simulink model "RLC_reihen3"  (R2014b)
settings: Solver=ode45  StartTime=0.0  StopTime=0.005  RelTol=1e-3
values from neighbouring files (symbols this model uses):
  ampl_ug = 2    [RLC_reihen_1.m]    (also in RLC_reihen_3.m; RLC_reihen_4.m)
  C = [0 1 0 0;0 0 0 1]    [impuls_antw_zustand_1.m]    (also in impuls_antwort_1.m = 1e-07; impuls_antwort_2.m = 1e-07; impuls_antwort_3.m = 1e-07; impuls_antwort_4.m = 1e-07)
  f_ug = 1000    [RLC_reihen_1.m]    (also in RLC_reihen_3.m; RLC_reihen_4.m)
  i0 = 0    [RLC_reihen_1.m]    (also in RLC_reihen_3.m; RLC_reihen_4.m)
  L = 0.01    [impuls_antwort_1.m]    (also in impuls_antwort_2.m; impuls_antwort_3.m; impuls_antwort_4.m; RLC_reihen_1.m)
  phi_ug = pi/3    (= 1.0471975512)    [RLC_reihen_1.m]    (also in RLC_reihen_3.m; RLC_reihen_4.m)
  R = 50    [impuls_antwort_1.m]    (also in impuls_antwort_2.m; impuls_antwort_3.m; impuls_antwort_4.m; RLC_reihen_1.m)
  uc0 = -2    [RLC_reihen_1.m]    (also in RLC_reihen_3.m; RLC_reihen_4.m)

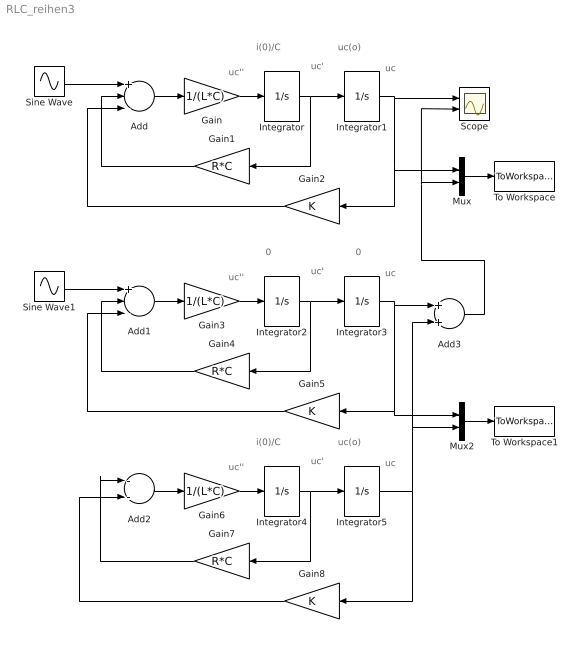
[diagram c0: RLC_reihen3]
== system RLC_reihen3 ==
  note: 0
  note: uc(o)
  note: i(0)/C
  note: uc''
  note: uc
  note: uc'
  note: 0
  note: uc''
  note: uc
  note: uc'
  note: uc(o)
  note: i(0)/C
  note: uc''
  note: uc
  note: uc'
  Add : Sum  Inputs=+--
  Add1 : Sum  Inputs=+--
  Add2 : Sum  Inputs=--
  Add3 : Sum
  Gain : Gain  Gain=1/(L*C)
  Gain1 : Gain  Gain=R*C
  Gain2 : Gain
  Gain3 : Gain  Gain=1/(L*C)
  Gain4 : Gain  Gain=R*C
  Gain5 : Gain
  Gain6 : Gain  Gain=1/(L*C)
  Gain7 : Gain  Gain=R*C
  Gain8 : Gain
  Integrator : Integrator  InitialCondition=i0/C
  Integrator1 : Integrator  InitialCondition=uc0
  Integrator2 : Integrator
  Integrator3 : Integrator
  Integrator4 : Integrator  InitialCondition=i0/C
  Integrator5 : Integrator  InitialCondition=uc0
  Mux : Mux  Inputs=2
  Mux2 : Mux  Inputs=2
  Scope : Scope  NumInputPorts=2
  Sine Wave : Sin  Amplitude=ampl_ug  Frequency=2*pi*f_ug  Phase=phi_ug  SampleTime=0
  Sine Wave1 : Sin  Amplitude=ampl_ug  Frequency=2*pi*f_ug  Phase=phi_ug  SampleTime=0
  To Workspace : ToWorkspace  VariableName=simout  SaveFormat=Timeseries  SampleTime=-1
  To Workspace1 : ToWorkspace  VariableName=simout1  SaveFormat=Timeseries  SampleTime=-1
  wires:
  Sine Wave/1 -> Add/1
  Add/1 -> Gain/1
  Gain/1 -> Integrator/1
  Integrator/1 -> Gain1/1, Integrator1/1
  Gain1/1 -> Add/2
  Gain2/1 -> Add/3
  Integrator1/1 -> Scope/1, Mux/1, Gain2/1
  Mux/1 -> To Workspace/1
  Sine Wave1/1 -> Add1/1
  Add1/1 -> Gain3/1
  Gain3/1 -> Integrator2/1
  Integrator2/1 -> Integrator3/1, Gain4/1
  Gain4/1 -> Add1/2
  Gain5/1 -> Add1/3
  Integrator3/1 -> Add3/1, Mux2/1, Gain5/1
  Add2/1 -> Gain6/1
  Gain6/1 -> Integrator4/1
  Integrator4/1 -> Gain7/1, Integrator5/1
  Integrator5/1 -> Mux2/2, Add3/2, Gain8/1
  Gain7/1 -> Add2/1
  Gain8/1 -> Add2/2
  Add3/1 -> Scope/2, Mux/2
  Mux2/1 -> To Workspace1/1
